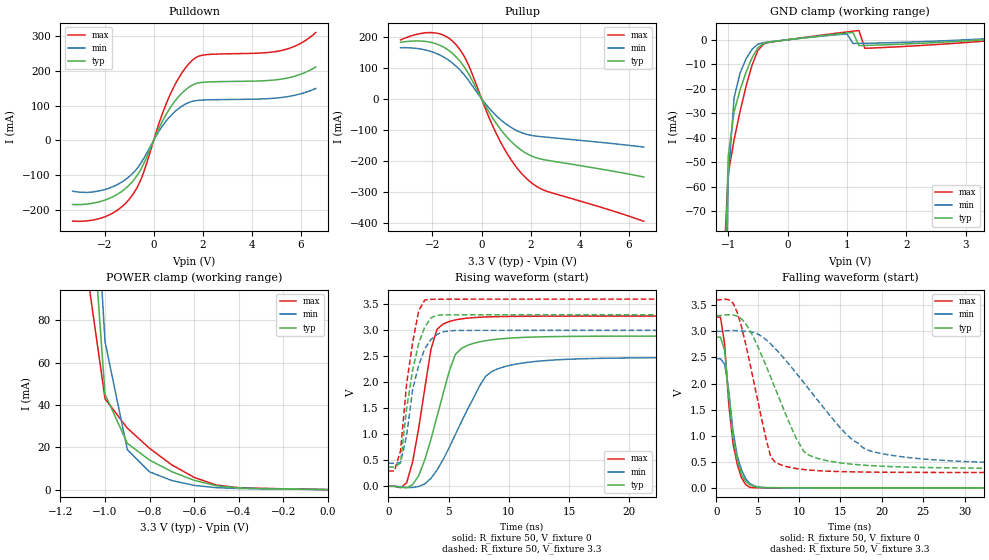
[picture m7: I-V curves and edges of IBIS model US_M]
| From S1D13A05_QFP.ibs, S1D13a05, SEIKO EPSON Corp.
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[Model]   US_M
Model_type I/O
Enable Active-Low
Polarity Non-Inverting
Vinh=2.0
Vinl=0.8
Vref=0
Vmeas=1.65
Rref=500
Cref=100pf
C_comp   5p   4p   6p
[Temperature Range] 25   85   -40
[Voltage Range]   3.3   3.0   3.6
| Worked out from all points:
|   slope of the pulldown table from 0 to 0.495 V, typ, clamps not added: 6.74 ohm
|   slope of the pullup table from 0 to 0.495 V, typ, clamps not added: 7.33 ohm
|   GND clamp passes 1 mA (typ) near -0.32 V on its own axis
|   POWER clamp passes 1 mA (typ) near -0.42 V on its own axis
|   falling waveform, R_fixture 50, V_fixture 0: 20-80 % time 1.29ns typ, 1.36ns min, 1.2ns max; typ from 2.89 V to 0 V
|   falling waveform, R_fixture 50, V_fixture 3.3: 20-80 % time 4.63ns typ, 8.03ns min, 2.72ns max; typ from 3.3 V to 0.372 V
|   rising waveform, R_fixture 50, V_fixture 0: 20-80 % time 2.09ns typ, 3.22ns min, 1.37ns max; typ from 0 V to 2.89 V
|   rising waveform, R_fixture 50, V_fixture 3.3: 20-80 % time 1.23ns typ, 1.28ns min, 1.04ns max; typ from 0.371 V to 3.3 V
[Pullup]
-3.3V     182mA      164.8mA    189.8mA
-2.6V     186.7mA    161.9mA    208.6mA
-2V       180.8mA    151.1mA    213.4mA
-1.5V     164.5mA    132.5mA    203.4mA
-1.1V     140.1mA    109.3mA    179.6mA
-600mV    89.77mA    66.62mA    120.5mA
300mV     -42.81mA   -29.74mA   -59.99mA
900mV     -111.5mA   -75.9mA    -158.2mA
1.5V      -159.1mA   -105.3mA   -229.4mA
2.1V      -187.1mA   -119.5mA   -275.7mA
2.7V      -199.1mA   -124.6mA   -300mA
6.6V      -252.7mA   -156.2mA   -395.8mA
[Pulldown]
-3.3V     -184.8mA   -146.4mA   -232.6mA
-1.9V     -169.9mA   -139.8mA   -217.7mA
-900mV    -121.6mA   -98.26mA   -161.1mA
-500mV    -80.82mA   -63.36mA   -109.6mA
300mV     47.55mA    35.72mA    66.22mA
700mV     96.96mA    71.67mA    136.6mA
1.1V      132.7mA    96.38mA    189.3mA
1.6V      160.5mA    113.3mA    232.8mA
2.1V      168.2mA    116.8mA    247mA
5.2V      176.9mA    123.8mA    259.4mA
5.9V      188.8mA    132.9mA    276.9mA
6.6V      211.7mA    149.8mA    311.1mA
[GND Clamp]
-3.3V     -5.924A    -5.017A    -7.449A
-1.1V     -152mA     -204.1mA   -104.9mA
-1V       -47.65mA   -57.62mA   -54.88mA
-900mV    -29.36mA   -23.57mA   -40.73mA
-700mV    -13.31mA   -7.844mA   -19.07mA
-500mV    -3.248mA   -1.813mA   -4.322mA
-300mV    -912uA     -812.9uA   -1.02mA
1V        2.756mA    2.383mA    3.2mA
1.1V      2.998mA    -1.533mA   3.495mA
1.2V      -2.385mA   -1.492mA   3.786mA
1.3V      -2.318mA   -1.447mA   -3.49mA
3.3V      1.036nA    369.4uA    -578.7uA
[POWER Clamp]
-3.3V     6.233A     5.277A     7.818A
-1.1V     192.1mA    248.4mA    117.4mA
-1V       45.09mA    69.85mA    42.92mA
-900mV    21.87mA    18.92mA    29.05mA
-800mV    13.93mA    8.361mA    19.47mA
-700mV    8.451mA    4.268mA    11.66mA
-600mV    4.382mA    1.988mA    5.75mA
-500mV    1.831mA    895.7uA    2.144mA
-400mV    789.2uA    527.7uA    899uA
0V        1.035nA    2.234nA    177.6pA
[Falling Waveform]
R_fixture=50
V_fixture=0
V_fixture_min=0
V_fixture_max=0
0s        2.889V     2.477V     3.274V
505.1ps   2.89V      2.477V     3.273V
1.01ns    2.64V      2.371V     2.756V
1.515ns   1.743V     1.861V     1.591V
2.02ns    954.6mV    1.096V     850.6mV
2.525ns   543.2mV    615.7mV    456.9mV
3.03ns    266.6mV    356.3mV    200.3mV
4.04ns    61.46mV    87.56mV    9.621mV
7.071ns   1.276mV    3.094mV    807.4uV
50ns      6.888uV    35.24uV    1.768uV
[Falling Waveform]
R_fixture=50
V_fixture=3.3
V_fixture_min=3.0
V_fixture_max=3.6
0s        3.3V       3V         3.6V
1.515ns   3.32V      3.015V     3.608V
2.525ns   3.294V     3.014V     3.369V
4.04ns    3.025V     2.995V     2.406V
6.566ns   2.128V     2.762V     603.1mV
7.576ns   1.729V     2.594V     457.6mV
10.61ns   693mV      2.011V     351mV
15.66ns   466mV      1.037V     309.4mV
18.69ns   426.3mV    704.9mV    302mV
50ns      372mV      450.9mV    294.6mV
[Rising Waveform]
R_fixture=50
V_fixture=0
V_fixture_min=0
V_fixture_max=0
0s        0V         0V         0V
1.515ns   -30.29mV   -24.34mV   64.45mV
2.525ns   207.3mV    -3.579mV   1.127V
3.535ns   902.7mV    151.6mV    2.633V
4.04ns    1.339V     310.8mV    3.02V
5.051ns   2.209V     743.3mV    3.169V
6.061ns   2.651V     1.238V     3.22V
8.081ns   2.8V       2.116V     3.257V
10.61ns   2.857V     2.35V      3.269V
50ns      2.889V     2.477V     3.274V
[Rising Waveform]
R_fixture=50
V_fixture=3.3
V_fixture_min=3.0
V_fixture_max=3.6
0s        371.4mV    443mV      294.5mV
505.1ps   371.4mV    443mV      294.5mV
1.01ns    445.7mV    456mV      680.4mV
1.515ns   1.491V     969.6mV    1.969V
2.02ns    2.239V     1.869V     2.77V
2.525ns   2.751V     2.33V      3.382V
3.03ns    3.066V     2.65V      3.585V
4.04ns    3.29V      2.922V     3.598V
5.556ns   3.298V     2.996V     3.599V
50ns      3.3V       3V         3.6V
[Ramp]
R_load=50
dV/dt_r   1.733E+0/2.052E-9   1.486E+0/3.179E-9   1.964E+0/1.328E-9
dV/dt_f   1.757E+0/4.623E-9   1.529E+0/8.025E-9   1.983E+0/2.709E-9
